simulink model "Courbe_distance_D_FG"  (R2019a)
settings: Solver=VariableStepAuto  StartTime=0.0  StopTime=6.283185307  MaxStep=0.001  RelTol=1e-6  SampleTimeConstraint=STIndependent

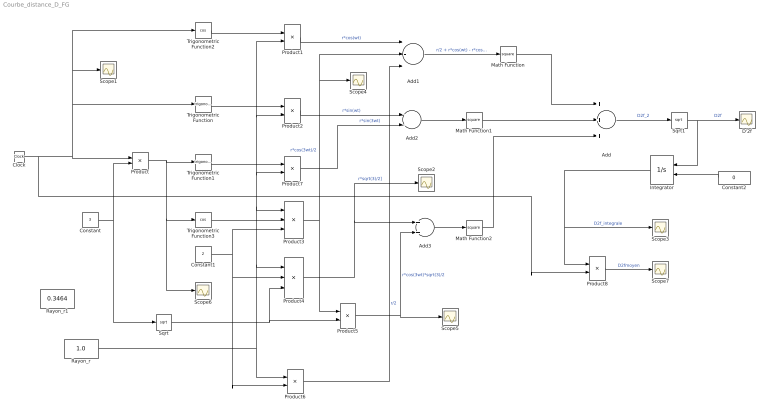
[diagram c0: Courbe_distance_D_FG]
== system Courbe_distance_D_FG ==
  Add : Sum  Inputs=+++
  Add1 : Sum  Inputs=+-+
  Add2 : Sum  Inputs=--
  Add3 : Sum
  Clock : Clock
  Constant : Constant  Value=3
  Constant1 : Constant  Value=2
  Constant2 : Constant  Value=0
  D'2f : Scope
  Integrator : Integrator  InitialConditionSource=external
  Math Function : Math  Operator=square
  Math Function1 : Math  Operator=square
  Math Function2 : Math  Operator=square
  Product{,1..2,5,7} (5 alike) : Product
  Product3 : Product  Inputs=**/
  Product4 : Product  Inputs=*/*
  Product6 : Product  Inputs=*/
  Product8 : Product  Inputs=*/
  Rayon_r : Constant  Value=1.0
  Rayon_r1 : Constant  Value=0.3464
  Scope{1..7} (7 alike) : Scope
  Sqrt : Sqrt
  Sqrt1 : Sqrt
  Trigonometric Function : Trigonometry
  Trigonometric Function1 : Trigonometry
  Trigonometric Function2 : Trigonometry  Operator=cos
  Trigonometric Function3 : Trigonometry  Operator=cos
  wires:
  Product/1 -> Scope6/1, Trigonometric Function3/1, Trigonometric Function1/1
  Constant/1 -> Product/2, Sqrt/1
  Clock/1 -> Product8/2, Trigonometric Function/1, Trigonometric Function2/1, Scope1/1, Product/1
  Trigonometric Function2/1 -> Product1/1
  Rayon_r/1 -> Product6/1, Product4/1, Product3/1, Product7/2, Product2/2, Product1/2
  Trigonometric Function/1 -> Product2/1
  Trigonometric Function3/1 -> Product3/2
  Constant1/1 -> Product6/2, Product4/2, Product3/3
  Sqrt/1 -> Product4/3, Product5/2
  Product3/1 -> Product5/1, Scope4/1, Add1/2  "r*cos(3wt)/2"
  Trigonometric Function1/1 -> Product7/1
  Product1/1 -> Add1/1  "r*cos(wt)"
  Product6/1 -> Add1/3  "r/2"
  Add1/1 -> Math Function/1  "r/2 + r*cos(wt) - r*cos(3wt)/2"
  Product2/1 -> Add2/1  "r*sin(wt)"
  Product7/1 -> Add2/2  "r*sin(3wt)"
  Add2/1 -> Math Function1/1
  Product4/1 -> Scope2/1, Add3/1  "r*sqrt(3)/2]"
  Add3/1 -> Math Function2/1
  Math Function/1 -> Add/1
  Math Function1/1 -> Add/2
  Math Function2/1 -> Add/3
  Product5/1 -> Add3/2, Scope5/1  "r*cos(3wt)*sqrt(3)/2"
  Add/1 -> Sqrt1/1  "D2f_2"
  Sqrt1/1 -> Integrator/1, D'2f/1  "D2f"
  Integrator/1 -> Scope3/1, Product8/1  "D2f_integrale"
  Constant2/1 -> Integrator/2
  Product8/1 -> Scope7/1  "D2fmoyen"
